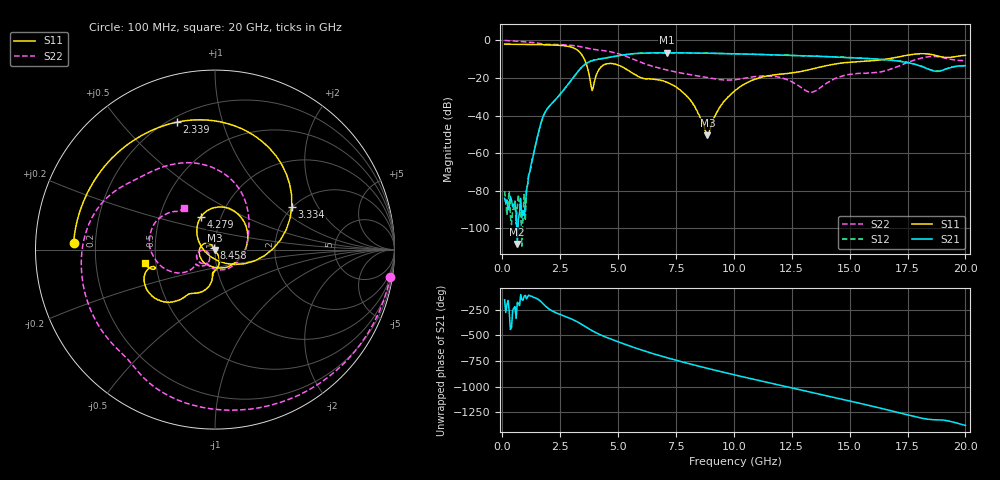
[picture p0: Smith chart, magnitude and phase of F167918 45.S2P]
!  2-Port S-parameters saved by WinCal
! VAR MeasName=S-Parameters (CALIBRATED_DATA) read from VNA (N5242A)
! VAR MeasDate=2016-11-22 10:26:58
! VAR NAME=F167918 45
! VAR FILENAME=F167918 45.S2P
! VAR DATE=2016-11-22 10:26:58
! VAR PHYS_PORTS=1,2
# Hz S DB R 50
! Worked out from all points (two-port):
!   401 points, 100 MHz to 20 GHz, reference 50 ohm
!   highest |S21| = -6.63 dB at 7.115 GHz (marker M1); lowest = -108.3 dB at 647.2 MHz (marker M2)
!   |S21| within 3 dB of the highest: 4.359 GHz to 15.67 GHz (11.31 GHz wide, 113 % of centre)
!   lowest |S11| = -50.6 dB at 8.856 GHz (marker M3), VSWR 1.01, Z = 49.7 - j0.155 ohm
!   |S11| at or under -10 dB: 3.54 GHz to 16.59 GHz (13.05 GHz wide, 130 % of centre)
!   |S22| runs from -27.6 to -0.1 dB; largest |S21 - S12| = 0.0054
!   S11 on the Smith chart (normalised r, x): 100 MHz: 0.12, +0.02; 2.339 GHz: 0.23, +0.72; 3.334 GHz: 1.98, +1.24; 4.279 GHz: 0.80, +0.31; 8.458 GHz: 0.99, +0.02; 20 GHz: 0.43, -0.08
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1e8  -2.07 177.3  -84.06 -154.3  -80.16 173.6  -0.10 -8.8
6.4725e8  -2.14 162.7  -108.32 -179.5  -87.81 -125.0  -0.49 -52.4
9.955e8  -2.20 153.2  -88.49 -110.3  -95.91 -105.1  -0.82 -77.8
1.74175e9  -2.36 130.3  -41.28 172.6  -41.21 172.0  -1.99 -124.3
2.33875e9  -2.60 106.7  -30.93 77.8  -30.93 77.4  -2.26 -152.3
3.33375e9  -6.20 29.2  -15.62 -20.5  -15.63 -20.5  -3.29 158.4
3.43325e9  -7.69 15.7  -14.30 -33.9  -14.31 -33.7  -3.55 153.6
3.881e9  -26.70 -123.1  -10.88 -95.0  -10.83 -95.1  -4.71 136.2
4.279e9  -13.99 112.7  -9.80 -139.0  -9.78 -139.3  -5.34 120.7
4.9755e9  -13.06 42.3  -8.28 159.3  -8.29 159.1  -7.03 88.2
5.72175e9  -18.11 -45.5  -7.06 99.1  -7.06 99.1  -10.40 54.2
6.7665e9  -21.08 -174.2  -6.65 24.5  -6.66 24.3  -14.80 11.4
7.11475e9  -22.34 161.4  -6.63 2.0  -6.65 1.9  -15.84 -6.4
8.458e9  -38.98 128.3  -6.79 -78.6  -6.79 -78.6  -19.01 -84.5
8.856e9  -50.60 -148.2  -6.87 -101.0  -6.87 -101.0  -19.82 -101.9
1.005e10  -26.72 -62.8  -7.18 -165.9  -7.20 -165.8  -20.98 -122.9
1.179125e10  -18.28 -92.0  -7.79 104.0  -7.77 104.1  -19.30 -160.0
1.338325e10  -15.28 -95.5  -8.38 23.1  -8.33 23.3  -27.62 -144.4
1.517425e10  -11.51 -114.1  -9.33 -68.0  -9.29 -68.1  -17.90 -135.3
1.67165e10  -9.76 -123.7  -10.48 -149.6  -10.46 -149.9  -15.61 -140.0
1.835825e10  -7.25 -155.1  -15.13 124.3  -14.99 123.6  -8.77 177.6
2e10  -7.98 -169.4  -13.54 63.1  -13.48 62.4  -10.77 126.1
